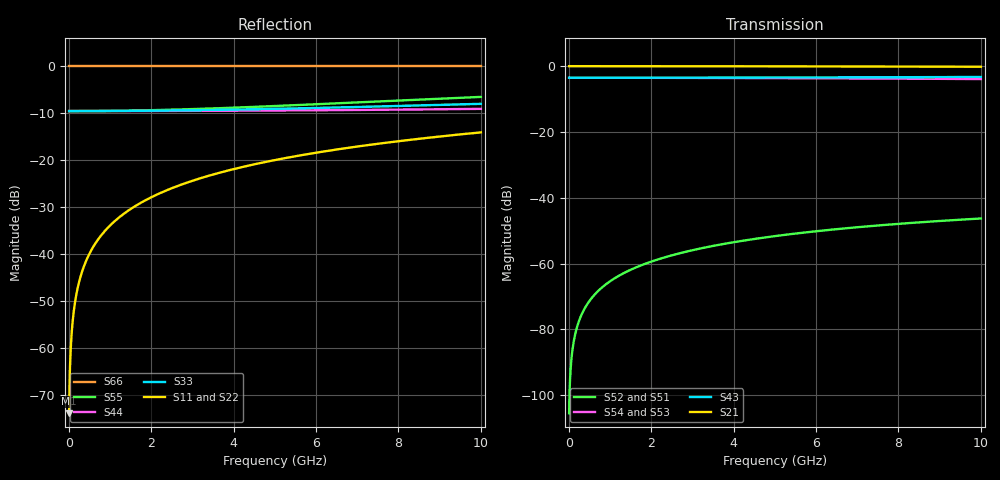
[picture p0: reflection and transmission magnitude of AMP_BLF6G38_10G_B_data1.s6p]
! Created Wed Jun 30 11:59:15 2010
# ghz S ma R 50
! 6 Port Network Data from SP1.SP block
! freq  magS11  angS11  magS12  angS12  magS13  angS13  magS14  angS14
!  magS15  angS15  magS16  angS16
!  magS21  angS21  magS22  angS22
!  magS23  angS23  magS24  angS24  magS25  angS25  magS26  angS26
!  magS31  angS31  magS32  angS32  magS33  angS33  magS34  angS34
!  magS35  angS35  magS36  angS36
!  magS41  angS41  magS42  angS42
!  magS43  angS43  magS44  angS44  magS45  angS45  magS46  angS46
!  magS51  angS51  magS52  angS52  magS53  angS53  magS54  angS54
!  magS55  angS55  magS56  angS56
!  magS61  angS61  magS62  angS62
!  magS63  angS63  magS64  angS64  magS65  angS65  magS66  angS66
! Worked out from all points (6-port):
!   1000 points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, 10 MHz to 10 GHz, reference 50 ohm
!   strongest paths, dB at 10 MHz, 2.51 GHz, 5.01 GHz, 7.51 GHz, 10 GHz:
!     S21: 0.0, 0.0, 0.0, -0.1, -0.2
!     S43: -3.5, -3.5, -3.5, -3.4, -3.3
!     S54: -3.5, -3.6, -3.6, -3.8, -3.9
!     S53: -3.5, -3.6, -3.7, -4.0, -4.3
!     S52: -105.5, -57.5, -51.6, -48.4, -46.3
!     S51: -105.5, -57.5, -51.6, -48.4, -46.3
!   lowest |S11| = -73.8 dB at 10 MHz (marker M1), VSWR 1.00, Z = 50 + j0.0202 ohm
!   |S11| at or under -10 dB: start of sweep to end of sweep
